| TEXAS INSTRUMENTS INCORPORATED
| Standard Linear and Logic Group
| IBIS Model of SN74ALVCH16827
| 20-BIT BUFFER/DRIVER WITH 3-STATE OUTPUTS
| This file contains package information for the following:
|  SSOP 56-pin (DL) package as [Component] ALVCH16827_DL
|  TSSOP 56-pin (DGG) package as [Component] ALVCH16827_DGG
| This device can be powered at the following Vccs:
|  1.8 volt Vcc
|  2.5 volt Vcc
|  3.3 volt Vcc
| This file provides unique models under the [Model Selector] for each Vcc.
| For operation at a specific Vcc, select the appropriate model after each
| [Model Selector] keyword.
[IBIS Ver]   3.2
[Comment char]  |_char
[File Name]   sn74alvch16827.ibs
[File Rev]   1.1 | a_die
[Date]   February 28, 2007
[Source]   Data created from TI-SPICE simulations at TI-SLL.
[Notes]   The following is an IBIS list for the SN74ALVCH16827.
   Please contact sllibis@ti.com with questions and
   comments concerning SLL IBIS models.
   This IBIS model is created from a BA (back annotated netlist)
   - FILE REV HISTORY
   - 1.1 Release IBIS file on 03/28/05
   - Non-monotonic data in ground-clamp due to bus-hold
[Disclaimer] Property of Texas Instruments Incorporated.  Unauthorized
   reproduction and/or distribution is strictly prohibited.
   This product is protected under copyright law.
   Created  2007, (C) Copyright  2007, Texas Instruments
   Incorporated, All Rights Reserved
   UNLESS THERE IS A SIGNED, WRITTEN AGREEMENT TO THE
   CONTRARY, TEXAS INSTRUMENTS (TI) IS PROVIDING THE IBIS
   MODELS  AND WITHOUT ANY WARRANTY, EXPRESSED OR
   IMPLIED.  TI assumes no liability for:
   1) the accuracy of the IBIS models provided to your
   company;
   2) the proper functioning of these IBIS Models in your
   design or for any resulting applications; or
   3) infringement of patents, copyrights or intellectual
   property rights resulting from your use of these IBIS
   models.
   TI provides IBIS Models as a service to our customers.
   You and your company shall not distribute, sell or give
   these models to anyone else without prior written
   permission from TI.
   TI reserves the right to make changes to our products or
   to discontinue any semiconductor product or service
   without notice, and advises our customers to obtain the
   latest version of relevant information to verify, before
   placing orders, that the information being relied on is
   current.
   Please be aware that your receipt and use of the IBIS
   information provided shall serve as acceptance of these
   terms and conditions.  If you do not accept these terms,
   you should return or destroy the IBIS models and any
   other accompanying information immediately.
| Component SN74ALVCH16827_DL 56-PIN SSOP
[Component]   SN74ALVCH16827_DL
[Manufacturer]   Texas Instruments, Inc.
[Package]
|   typ   min   max
R_pkg   5.500e-02   4.800e-02   6.700e-02
L_pkg   6.539e-09   4.803e-09   9.746e-09
C_pkg   8.570e-13   5.000e-13   1.351e-12
[Pin]   signal_name   model_name   R_pin   L_pin   C_pin
1   1NOE1   ALVCH16827_NOE   6.400e-02   9.646e-09   1.202e-12
2   1Y1   ALVCH16827_OUT   5.900e-02   8.723e-09   1.348e-12
3   1Y2   ALVCH16827_OUT   5.900e-02   8.139e-09   1.223e-12
4   GND   GND   5.600e-02   7.554e-09   1.088e-12
5   1Y3   ALVCH16827_OUT   5.400e-02   6.991e-09   9.660e-13
6   1Y4   ALVCH16827_OUT   5.300e-02   6.659e-09   9.730e-13
7   VCC   POWER   5.500e-02   6.321e-09   9.050e-13
8   1Y5   ALVCH16827_OUT   5.600e-02   5.942e-09   7.130e-13
9   1Y6   ALVCH16827_OUT   5.700e-02   5.768e-09   6.780e-13
10   1Y7   ALVCH16827_OUT   5.400e-02   5.459e-09   6.310e-13
11   GND   GND   5.100e-02   5.224e-09   6.380e-13
12   1Y8   ALVCH16827_OUT   4.800e-02   5.088e-09   6.010e-13
13   1Y9   ALVCH16827_OUT   5.000e-02   5.021e-09   5.180e-13
14   1Y10   ALVCH16827_OUT   5.100e-02   4.803e-09   5.000e-13
15   2Y1   ALVCH16827_OUT   5.100e-02   4.803e-09   5.000e-13
16   2Y2   ALVCH16827_OUT   5.000e-02   5.021e-09   5.180e-13
17   2Y3   ALVCH16827_OUT   4.800e-02   5.088e-09   6.010e-13
18   GND   GND   5.100e-02   5.224e-09   6.380e-13
19   2Y4   ALVCH16827_OUT   5.400e-02   5.459e-09   6.310e-13
20   2Y5   ALVCH16827_OUT   5.700e-02   5.768e-09   6.770e-13
21   2Y6   ALVCH16827_OUT   5.500e-02   5.942e-09   7.150e-13
22   VCC   POWER   5.500e-02   6.321e-09   9.070e-13
23   2Y7   ALVCH16827_OUT   5.300e-02   6.659e-09   9.720e-13
24   2Y8   ALVCH16827_OUT   5.400e-02   6.991e-09   9.660e-13
25   GND   GND   5.600e-02   7.554e-09   1.087e-12
26   2Y9   ALVCH16827_OUT   5.900e-02   8.139e-09   1.223e-12
27   2Y10   ALVCH16827_OUT   5.900e-02   8.727e-09   1.351e-12
28   2NOE1   ALVCH16827_NOE   6.700e-02   9.746e-09   1.210e-12
29   2NOE2   ALVCH16827_NOE   6.300e-02   9.630e-09   1.203e-12
30   2A10   ALVCH16827_IN   6.000e-02   8.751e-09   1.349e-12
31   2A9   ALVCH16827_IN   6.000e-02   8.184e-09   1.224e-12
32   GND   GND   5.600e-02   7.543e-09   1.087e-12
33   2A8   ALVCH16827_IN   5.400e-02   7.005e-09   9.690e-13
34   2A7   ALVCH16827_IN   5.600e-02   6.714e-09   9.750e-13
35   VCC   POWER   5.800e-02   6.384e-09   9.090e-13
36   2A6   ALVCH16827_IN   5.700e-02   5.976e-09   7.170e-13
37   2A5   ALVCH16827_IN   5.700e-02   5.743e-09   6.770e-13
38   2A4   ALVCH16827_IN   5.400e-02   5.468e-09   6.310e-13
39   GND   GND   5.500e-02   5.329e-09   6.440e-13
40   2A3   ALVCH16827_IN   5.200e-02   5.189e-09   6.060e-13
41   2A2   ALVCH16827_IN   5.200e-02   5.053e-09   5.190e-13
42   2A1   ALVCH16827_IN   5.200e-02   4.825e-09   5.020e-13
43   1A10   ALVCH16827_IN   5.400e-02   4.897e-09   5.060e-13
44   1A9   ALVCH16827_IN   5.200e-02   5.093e-09   5.210e-13
45   1A8   ALVCH16827_IN   5.100e-02   5.179e-09   6.080e-13
46   GND   GND   5.400e-02   5.314e-09   6.450e-13
47   1A7   ALVCH16827_IN   5.500e-02   5.511e-09   6.320e-13
48   1A6   ALVCH16827_IN   5.700e-02   5.770e-09   6.770e-13
49   1A5   ALVCH16827_IN   5.600e-02   5.956e-09   7.160e-13
50   VCC   POWER   5.500e-02   6.320e-09   9.050e-13
51   1A4   ALVCH16827_IN   5.200e-02   6.621e-09   9.680e-13
52   1A3   ALVCH16827_IN   5.300e-02   6.974e-09   9.660e-13
53   GND   GND   5.700e-02   7.571e-09   1.089e-12
54   1A2   ALVCH16827_IN   5.700e-02   8.097e-09   1.219e-12
55   1A1   ALVCH16827_IN   5.900e-02   8.723e-09   1.349e-12
56   1NOE2   ALVCH16827_NOE   6.100e-02   9.560e-09   1.199e-12
| Component SN74ALVCH16827_DGG 56-PIN TSSOP
[Component]   SN74ALVCH16827_DGG
[Manufacturer]   Texas Instruments, Inc.
[Package]
|   typ   min   max
R_pkg   5.400e-02   4.000e-02   8.300e-02
L_pkg   3.546e-09   2.838e-09   5.045e-09
C_pkg   5.580e-13   4.120e-13   7.380e-13
[Pin]   signal_name   model_name   R_pin   L_pin   C_pin
1   1NOE1   ALVCH16827_NOE   7.600e-02   5.003e-09   7.120e-13
2   1Y1   ALVCH16827_OUT   7.600e-02   4.539e-09   7.230e-13
3   1Y2   ALVCH16827_OUT   8.300e-02   4.357e-09   7.080e-13
4   GND   GND   4.200e-02   3.999e-09   6.830e-13
5   1Y3   ALVCH16827_OUT   4.200e-02   3.806e-09   6.700e-13
6   1Y4   ALVCH16827_OUT   4.300e-02   3.603e-09   6.160e-13
7   VCC   POWER   4.400e-02   3.440e-09   5.520e-13
8   1Y5   ALVCH16827_OUT   4.600e-02   3.306e-09   5.090e-13
9   1Y6   ALVCH16827_OUT   4.700e-02   3.194e-09   4.820e-13
10   1Y7   ALVCH16827_OUT   4.800e-02   3.088e-09   4.630e-13
11   GND   GND   5.000e-02   2.987e-09   4.350e-13
12   1Y8   ALVCH16827_OUT   5.100e-02   2.910e-09   4.230e-13
13   1Y9   ALVCH16827_OUT   5.200e-02   2.894e-09   4.220e-13
14   1Y10   ALVCH16827_OUT   5.300e-02   2.840e-09   4.220e-13
15   2Y1   ALVCH16827_OUT   5.300e-02   2.850e-09   4.230e-13
16   2Y2   ALVCH16827_OUT   5.200e-02   2.886e-09   4.210e-13
17   2Y3   ALVCH16827_OUT   5.100e-02   2.883e-09   4.190e-13
18   GND   GND   5.000e-02   2.941e-09   4.300e-13
19   2Y4   ALVCH16827_OUT   4.900e-02   3.031e-09   4.570e-13
20   2Y5   ALVCH16827_OUT   4.700e-02   3.131e-09   4.760e-13
21   2Y6   ALVCH16827_OUT   4.600e-02   3.244e-09   5.030e-13
22   VCC   POWER   4.400e-02   3.387e-09   5.500e-13
23   2Y7   ALVCH16827_OUT   4.300e-02   3.566e-09   6.320e-13
24   2Y8   ALVCH16827_OUT   4.200e-02   3.801e-09   6.870e-13
25   GND   GND   4.100e-02   3.961e-09   6.870e-13
26   2Y9   ALVCH16827_OUT   8.100e-02   4.291e-09   7.110e-13
27   2Y10   ALVCH16827_OUT   7.600e-02   4.561e-09   7.380e-13
28   2NOE1   ALVCH16827_NOE   7.500e-02   5.045e-09   7.240e-13
29   2NOE2   ALVCH16827_NOE   7.300e-02   5.020e-09   7.140e-13
30   2A10   ALVCH16827_IN   7.400e-02   4.532e-09   7.200e-13
31   2A9   ALVCH16827_IN   8.300e-02   4.336e-09   7.080e-13
32   GND   GND   4.000e-02   3.957e-09   6.840e-13
33   2A8   ALVCH16827_IN   4.200e-02   3.789e-09   6.800e-13
34   2A7   ALVCH16827_IN   4.300e-02   3.540e-09   6.240e-13
35   VCC   POWER   4.400e-02   3.361e-09   5.460e-13
36   2A6   ALVCH16827_IN   4.600e-02   3.222e-09   4.980e-13
37   2A5   ALVCH16827_IN   4.700e-02   3.110e-09   4.710e-13
38   2A4   ALVCH16827_IN   4.800e-02   3.012e-09   4.510e-13
39   GND   GND   5.000e-02   2.934e-09   4.230e-13
40   2A3   ALVCH16827_IN   5.100e-02   2.879e-09   4.120e-13
41   2A2   ALVCH16827_IN   5.200e-02   2.883e-09   4.130e-13
42   2A1   ALVCH16827_IN   5.300e-02   2.847e-09   4.170e-13
43   1A10   ALVCH16827_IN   5.300e-02   2.838e-09   4.170e-13
44   1A9   ALVCH16827_IN   5.200e-02   2.887e-09   4.160e-13
45   1A8   ALVCH16827_IN   5.100e-02   2.897e-09   4.160e-13
46   GND   GND   5.000e-02   2.965e-09   4.270e-13
47   1A7   ALVCH16827_IN   4.800e-02   3.047e-09   4.550e-13
48   1A6   ALVCH16827_IN   4.700e-02   3.138e-09   4.740e-13
49   1A5   ALVCH16827_IN   4.600e-02   3.250e-09   5.030e-13
50   VCC   POWER   4.400e-02   3.390e-09   5.500e-13
51   1A4   ALVCH16827_IN   4.300e-02   3.546e-09   6.260e-13
52   1A3   ALVCH16827_IN   4.200e-02   3.783e-09   6.860e-13
53   GND   GND   4.000e-02   3.955e-09   6.820e-13
54   1A2   ALVCH16827_IN   8.300e-02   4.330e-09   7.010e-13
55   1A1   ALVCH16827_IN   7.700e-02   4.562e-09   7.240e-13
56   1NOE2   ALVCH16827_NOE   7.500e-02   5.029e-09   7.120e-13
| Model ALVCH16827_IN
[Model Selector]   ALVCH16827_IN
ALVCH16827_IN_18   1.8 volt Vcc
ALVCH16827_IN_25   2.5 volt Vcc
ALVCH16827_IN_33   3.3 volt Vcc
| Model ALVCH16827_NOE
[Model Selector]   ALVCH16827_NOE
ALVCH16827_NOE_18   1.8 volt Vcc
ALVCH16827_NOE_25   2.5 volt Vcc
ALVCH16827_NOE_33   3.3 volt Vcc
| Model ALVCH16827_OUT
[Model Selector]   ALVCH16827_OUT
ALVCH16827_OUT_18   1.8 volt Vcc
ALVCH16827_OUT_25   2.5 volt Vcc
ALVCH16827_OUT_33   3.3 volt Vcc
| Models and submodels in the file (9): ALVCH16827_IN_18 (Input), ALVCH16827_IN_25 (Input), ALVCH16827_IN_33 (Input), ALVCH16827_NOE_18 (Input), ALVCH16827_NOE_25 (Input), ALVCH16827_NOE_33 (Input), ALVCH16827_OUT_18 (3-state), ALVCH16827_OUT_25 (3-state), ALVCH16827_OUT_33 (3-state)
